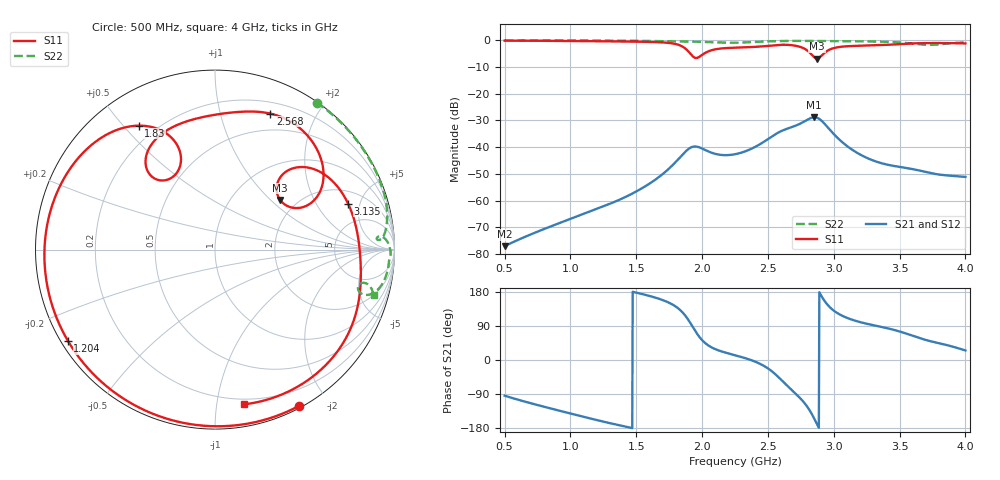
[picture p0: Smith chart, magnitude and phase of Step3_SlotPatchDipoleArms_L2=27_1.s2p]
! TOUCHSTONE file generated by CST MICROWAVE STUDIO
! Date and time: Mon May 18 03:45:28 2020
! Project name: DualBand_DualMode_Antenna_FD_SteppedDesign.cst
! Parameters = {FPL=20; FPW=20; L=50; ST=10; SW=30; W=52; WF=7; ext=10; gap=1; inset=13}
! Header version: 2015
! Port assignment regex: !\s*Touchstone port\s*([0-9]+)\s*=\s*CST MWS port\s*([0-9]+)\s*\(\"(.*)\"\)(\s*mode\s*([0-9]+))?.*
! Touchstone port assignment:
! Touchstone port 1 = CST MWS port 1 ("")
! Touchstone port 2 = CST MWS port 2 ("")
# GHz S MA R 50
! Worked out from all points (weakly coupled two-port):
!   1006 points, 500 MHz to 4 GHz, reference 50 ohm
!   highest |S21| = -28.80 dB at 2.852 GHz (marker M1); lowest = -77.1 dB at 500 MHz (marker M2)
!   lowest |S11| = -6.8 dB at 2.873 GHz (marker M3), VSWR 2.68, Z = 82.2 + j57.3 ohm
!   |S11| at or under -10 dB: nowhere
!   |S22| runs from -1.7 to 0.0 dB; largest |S21 - S12| = 7.1e-06
!   S11 on the Smith chart (normalised r, x): 500 MHz: 0.02, -1.68; 1.204 GHz: 0.02, -0.28; 1.83 GHz: 0.14, +0.55; 2.568 GHz: 0.31, +1.44; 3.135 GHz: 2.91, +3.87; 4 GHz: 0.16, -1.20
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0.5  0.9886 -61.6  0.0001398 -94.1  0.0001398 -94.0  0.9963 55.3
0.787  0.9824 -96.9  0.0002846 -122.2  0.0002842 -122.3  0.997 34.7
1.0845  0.97 -133.6  0.0005427 -148.6  0.0005434 -148.8  0.9955 22.8
1.2035  0.9644 -148.2  0.0007014 -158.8  0.0006987 -159.1  0.9934 19.3
1.4485  0.9507 -179.0  0.00127 -178.1  0.00127 -178.0  0.9843 13.3
1.669  0.9244 150.7  0.002721 161.9  0.002721 161.9  0.9704 9.1
1.83  0.8112 121.6  0.006351 132.9  0.00635 132.9  0.9576 6.6
1.907  0.5774 109.7  0.009618 99.7  0.009618 99.7  0.9498 5.5
1.977  0.4888 128.0  0.00996 62.0  0.00996 62.0  0.9411 4.6
2.068  0.6499 126.0  0.007937 34.1  0.007938 34.1  0.9266 3.6
2.25  0.7299 103.8  0.007371 12.7  0.007371 12.7  0.9037 4.0
2.5685  0.818 67.9  0.01816 -41.4  0.01816 -41.4  0.9693 1.6
2.7365  0.7661 38.7  0.02692 -97.7  0.02692 -97.7  0.9787 -1.6
2.8345  0.5332 26.0  0.03572 -143.4  0.03572 -143.4  0.973 -3.3
2.852  0.4821 29.3  0.03632 -154.9  0.03632 -154.9  0.9721 -3.6
2.873  0.4563 37.2  0.03561 -169.3  0.03562 -169.3  0.9715 -3.8
2.971  0.6761 42.9  0.02112 139.1  0.02112 139.1  0.9709 -5.3
3.1355  0.7845 19.0  0.009109 106.8  0.009109 106.8  0.9659 -8.0
3.419  0.829 -11.6  0.004635 82.8  0.004634 82.9  0.9363 -13.6
3.664  0.8871 -39.6  0.003589 56.6  0.003586 56.7  0.8383 -16.3
3.8215  0.892 -58.5  0.003023 42.5  0.003024 42.5  0.8515 -12.6
4  0.8772 -79.3  0.002772 25.2  0.002772 25.2  0.9193 -16.1
